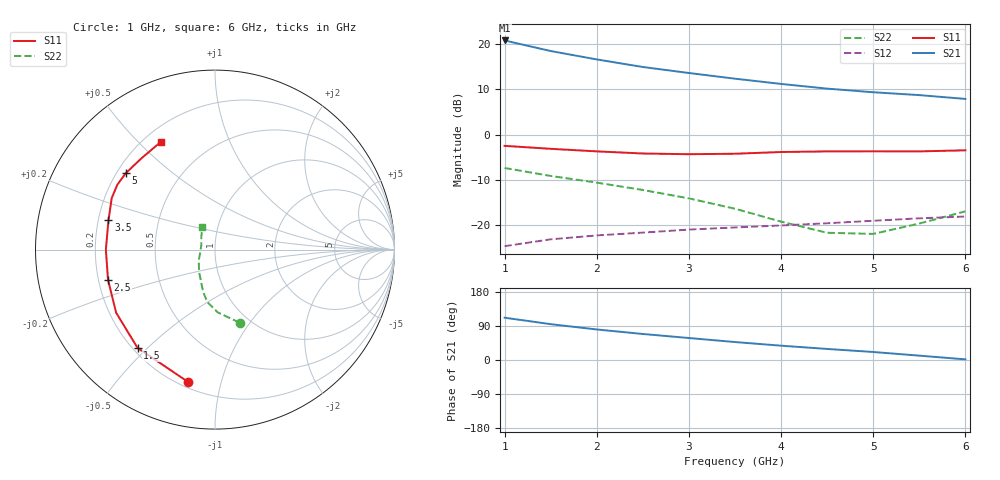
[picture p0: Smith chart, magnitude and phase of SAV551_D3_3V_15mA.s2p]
! Created Mon Oct 27 14:24:48 2008
# hz S ma R 50
! 2 Port Network Data from SP1.SP block
! freq  magS11  angS11  magS21  angS21  magS12  angS12  magS22  angS22
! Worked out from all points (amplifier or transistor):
!   11 points, 1 GHz to 6 GHz, reference 50 ohm
!   highest |S21| = 20.7 dB at 1 GHz (marker M1)
!   |S21| within 3 dB of that: start of sweep to 1.681 GHz
!   unconditionally stable (mu >= 1): 4.705 GHz to end of sweep
!   at 1.5 GHz: K = 0.45, MSG = 20.7 dB, |S12| = -23.1 dB
!   at 3.5 GHz: K = 0.88, MSG = 16.4 dB, |S12| = -20.5 dB
!   at 6 GHz: K = 1.07, MAG = 11.3 dB, |S12| = -18.0 dB
!   S11 on the Smith chart (normalised r, x): 1 GHz: 0.23, -0.79; 1.5 GHz: 0.22, -0.47; 2.5 GHz: 0.24, -0.13; 3.5 GHz: 0.24, +0.13; 5 GHz: 0.24, +0.35; 6 GHz: 0.27, +0.58
1e9  0.7519 -101.6  10.89 111.6  0.05903 39.1  0.429 -71.4
1.5e9  0.6972 -128.2  8.329 94.5  0.07023 30.6  0.3504 -87.4
2e9  0.6536 -147.4  6.73 80.6  0.07751 24.8  0.2958 -98.3
2.5e9  0.6192 -164.3  5.555 68.7  0.08329 20.5  0.2454 -105.5
3e9  0.608 -179.9  4.769 58.0  0.0899 17.0  0.1984 -112.8
3.5e9  0.6155 164.7  4.129 47.4  0.0949 13.3  0.1526 -125.4
4e9  0.643 153.5  3.616 37.8  0.09982 10.0  0.11 -145.7
4.5e9  0.6531 146.5  3.209 29.2  0.1055 7.2  0.08291 -171.2
5e9  0.6545 139.5  2.928 21.2  0.1124 4.0  0.08056 161.2
5.5e9  0.6532 128.8  2.723 11.5  0.1197 -0.3  0.1048 136.5
6e9  0.6714 116.8  2.472 1.7  0.1252 -4.4  0.1428 119.7
